(* Logix 5000 AddOnInstructionDefinition export PPD_IO_Link_Cyclic_Com_1_0_0; software revision 35.00 *)

ADD_ON_INSTRUCTION PPD_IO_Link_Cyclic_Com_1_0_0   (* revision 1.0 0, ExecutePrescan, ExecuteEnableInFalse *)
// FUNCTION_BLOCK PPD IO-Link Allen Breadley
VAR_INPUT
   in_b_RELEASE_FUNCTION_BLOCK : BOOL; {visible}
   in_b_00_FAST_STOP : BOOL; {visible}
   in_b_02_ACKNOLEDGE : BOOL; {visible}
   in_b_06_REPEAT_COMMAND_TOGGLE : BOOL; {visible}
   in_b_07_GRIP_DIRECTION : BOOL; {visible}
   in_b_08_JOG_MODE_NEGATIVE : BOOL; {visible}
   in_b_09_JOG_MODE_POSITIVE : BOOL; {visible}
   in_b_10_EXHAUST : BOOL; {visible}
   in_b_11_CALIBRATE : BOOL; {visible}
   in_b_16_MOVE_TO_ABSOLUTE_POSITION : BOOL; {visible}
   in_b_17_MOVE_TO_RELATIVE_POSITION : BOOL; {visible}
   in_b_18_FULLY_CLOSE : BOOL; {visible}
   in_b_19_FULLY_OPEN : BOOL; {visible}
   in_b_20_GRIP_WORKPIECE : BOOL; {visible}
   in_b_21_GRIP_WORKPIECE_AT_EXPECTED_POS : BOOL; {visible}
   in_b_22_CLOSE_ALL_VALVES : BOOL; {visible}
   in_usi_GAIN : USINT; {visible}
   in_usi_SPEED : USINT; {visible}
   in_ui_TARGET_POSITION_PRECICION : UINT; {visible}
   in_di_TARGET_POSITION : DINT; {visible}
   in_ui_TARGET_PRESSURE : UINT; {visible}
END_VAR
VAR_OUTPUT
   out_b_00_READY_FOR_OPERATION : BOOL; {access Read Only, visible}
   out_b_01_CONTOL_AUTHORITY_FIELDBUS : BOOL; {access Read Only, visible}
   out_b_03_NOT_FEASIBLE : BOOL; {access Read Only, visible}
   out_b_04_SENSOR_CALIBRATED : BOOL; {access Read Only, visible}
   out_b_05_COMMAND_RECEIVED_TOGGLE : BOOL; {access Read Only, visible}
   out_b_06_WARNING : BOOL; {access Read Only, visible}
   out_b_07_ERROR : BOOL; {access Read Only, visible}
   out_b_08_ALL_VALVES_CLOSED : BOOL; {access Read Only, visible}
   out_b_09_EXHAUSTED : BOOL; {access Read Only, visible}
   out_b_16_POSITION_REACHED : BOOL; {access Read Only, visible}
   out_b_17_NO_WORKPIECE_DETECTED : BOOL; {access Read Only, visible}
   out_b_18_WORKPIECE_GRIPPED : BOOL; {access Read Only, visible}
   out_b_19_WRONG_WORKPIECE_GRIPPED : BOOL; {access Read Only, visible}
   out_b_20_WORKPIECE_LOST : BOOL; {access Read Only, visible}
   out_usi_WARNING_CODE : USINT; {access Read Only, visible}
   out_usi_ERROR_CODE : USINT; {access Read Only, visible}
   out_di_ACTUAL_POSITION : DINT; {access Read Only, visible}
   out_i_ACTUAL_PRESSURE : INT; {access Read Only, visible}
END_VAR
VAR_IN_OUT
   in_PPD_PROZESS_DATA_IN : AB:PPD_XX_A4AF20E5:I:0; {required}
   out_PPD_PROZESS_DATA_OUT : AB:PPD_XX_88C23E22:O:0; {required}
END_VAR

ROUTINE EnableInFalse   (* structured text *)
   //////////////////////////////////////////////////////////////
   //   Copyright (c)  <Company Information>
   //--------------------------------------------------------------
   //   Routine: <Routine Name>
   //       Author: <Developer Name>
   //   Created: <Date>
   //--------------------------------------------------------------
   //   Description:
   //
   //   History:
   //
   /////////////////////////////////////////////////////////////
END_ROUTINE

ROUTINE Logic   (* structured text *)
   
   (*
   FUNCTION_BLOCK FB_SFP_EGU/EGK Allen Breadley
   TITLE = 'PPD_Cyclic_Communication'
   VERSION : '1.0.0'
   AUTHOR  : 'SCHUNK'
   NAME    : 'PPD_Cyclic_Communication'
   FAMILY  : 'SCHUNK'
   Used Products : PPD
   Projekt Nr.:
   =============================================================================
    Schunk GmbH&Co.KG
    (c)Copyright (2022) All Rights Reserved
   -----------------------------------------------------------------------------
    Library:       Schunk
    Tested with:   V35.00.00
                   Schunk FW release 5.x
    Engineering:   Studio 5000 V35.00.00
    Restrictions:  XXX(OB types, etc.)
    Requirements:  (hardware, technological package, memory needed, etc.)
    Functionality: The Funktion Block communicates Cyclic with the Gripper to read and wright Data
   
   *************************************************************************
   Historie
   
   ####################
   1.0.0
   Release Funktion Block
   TagType="Base" DataType="BOOL" Usage="Input" Radix="Binary" Required="false" Visible="true" ExternalAccess="Read Only"
   
   *************************************************************************)
   	(*English
   
       Statement section REGION
   
       *************************************************************************
       The function block is TO read AND transfer cyclic parameters that are changed FOR specific functions in the device
       can be used TO make The application process safer OR faster.
   
       Input parameters:
       ------------------
       b_RELEASE_FUNCTION_BLOCK            : Release FOR processing the block
   
       b_00_FAST_STOP                      : immediate shutdown of The process currently running in the gripper and shutdown of the motor phases
       b_02_ACKNOLEDGE                     : As long as the PPD is in error state and if an acknowledge was triggered, the PPD shall check if there are still any error causes.
                                             If there are no error causes any more, the state shall change to operational.
                                             Operational readiness is not established (again).
                                             If there are still any error causes, the status shall remain in error state and transmit the latest error code.
       b_06_REPEAT_COMMAND_TOGGLE          : The command that is still pending can, if it is a repeatable command, be repeated without loss OF Time for each positive and negative change of this bit
       b_07_GRIP_DIRECTION                 : determines The gripping direction. FALSE = external gripping (the workpiece is gripped from the outside) / True = internal gripping (the workpiece is gripped from the inside).
   
       b_08_JOG_MODE_NEGATIVE              : The gripper shall execute a movement with a fix velocity in the control bit corresponding direction.
                                             The value of the used fix velocity shall be 1 mm/s.
                                             Negative means a movement in the direction of decreasing position values. Function is also possible without "Calibration".
       b_09_JOG_MODE_POSITIVE              : The gripper shall execute a movement with a fix velocity in the control bit corresponding direction.
                                             The value of the used fix velocity shall be 1 mm/s.
                                             Positive means a movement in the direction of increasing position values. Function is also possible without "Calibration".
       b_10_EXHAUST                        : As soon as this function has been triggered the PPD shall open all valves to exhaust the air of both chambers.
                                             To trigger this function the PPD shall be in operation or error status.
       b_11_CALIBRATE                      : The calibrate function creates a routine in the PPD that determines the minimum and maximum position of the connected pneumatic product,
                                             provided a measuring system is available. The routine runs automatically.
   
       b_16_MOVE_TO_ABSOLUTE_POSITION      : When executing the command, the PPD tries to move to the specified position "Tag Position".
                                             In order to be able to execute this function, further parameters must be transferred: target accuracy, speed, gain.
       b_17_MOVE_TO_RELATIVE_POSITION      : When the command is executed, the PPD attempts to move to the specified, calculated position.
                                             In order to be able to execute this function, further parameters must be transferred: target position, target accuracy, speed, gain.
       b_18_FULLY_CLOSE                    : With this function, the PPD executes a movement to the minimum possible position.
       b_18_FULLY_OPEN                     : With this function, the PPD executes a movement to the maximum possible position.
       b_20_GRIP_WORKPIECE                 : The gripper shall grip workpieces at a nonspecific position.
                                             To execute this function the following parameter values shall be transmitted.
                                                   - target pressure difference
                                                   - speed
                                                   - grip direction (control bit)
       b_21_GRIP_WORKPIECE_AT_EXPECTED_POSITION : The gripper should grip workpieces at a specific position.
                                                  To execute this function, the following parameter values must be transferred.
                                                        - target position
                                                        - target pressure difference
                                                        - speed
       b_22_CLOSE_ALL_VALVES               : As soon as this function has been triggered the PPD shall close all valves.
   
       usi_GAIN                            : If a function needs a gain value to execute, the IO-Link master must transfer this value in the cyclic gain parameter.
                                             The gain value ranges from 1 to 10
       usi_SPEED                           : If a function needs a speed value to execute, the IO-Link-Master shall transmit this value in the cyclic parameter speed.
                                             Valid values shall be 1 to 10.
       i_TARGET_POSITION_PRECICION         : The parameter must represent a value in micrometers [µm].
                                             Valid values are between 500 µm and 15,000 µm.
       di_TARGET_POSITION                  : Valid values shall be -5.000.000 µm to 5.000.000 µm.
       ui_TARGET_PRESSURE			        : The target pressure difference shall represent the mathematical absolute value of the pressure difference between the two compression chambers.
                                             Valid values shall be 2000 mbar to 8.000 mbar.
   
       #################
   
   
   
       Output parameters:
       ------------------
   
       b_00_READY_FOR_OPERATION            : indicates that the gripper is ready FOR operation
       b_01_CONTOL_AUTHORITY_FIELDBUS      : indicates whether the fieldbus has control authority over the gripper
       b_03_NOT_FEASIBLE                   : Indicates that the last issued command cannot be executed.
                                               Possible causes are:
                                               - a new command was sent although the command that is still active has NOT yet been processed.
                                               - 2 OR more control commands simultaneously active in the control word
                                               - Parameter data FOR position, speed OR force are outside the permissible limits.
   
       b_04_SENSOR_CALIBRATED              : indicates that the "Calibrate" command was executed correctly and the sensor is calibrated
       b_05_COMMAND_RECEIVED_TOGGLE        : indicates that a command was sent to The gripper via the bus. the command does not have TO be processed or started at the time it is displayed.
       b_06_WARNING                        : signals a warning in the gripper, e.g. temperature warning
       b_07_ERROR                          : signals a fault in the gripper, e.g. rapid stop
       b_08_ALL_VALVES_CLOSED              : indicates that all Valves are closed
       b_09_EXHAUSTED                      : indicates that the EXHAUST funktion is completed successfully
   
       b_16_POSITION_REACHED               : signals that the relative or absolute position has been approached
       b_17_NO_WORKPIECE_DETECTED          : indicates that no workpiece was detected
       b_18_WORKPIECE_GRIPPED              : signals that a workpiece has been gripped
       b_19_WRONG_WORKPIECE_DETECTED       : signals that a wrong workpiece was detected
       b_20_WORKPIECE_LOST                 : signals that the gripped workpiece was lost
   
       usi_WARNING_CODE                     : Output of the gripper's warning code
       usi_ERROR_CODE                       : Output of the error code of the gripper
   
       di_ACTUAL_POSITION                  : the current position OF The gripper is returned here
       i_ACTUAL_PRESSURE_DIFFERENCE        : As long as a workpiece is being gripped, the IO-Link master should be able to evaluate the actual signed pressure difference value by reading out the cyclic parameter actual pressure difference.
                                             The value is shown in millibar [mbar].
   
       *************************************************************************)
   
   
   (*************************************************************************
       Der Baustein soll Zyklische Parameter einlesen und übertragen, welche für bestimmte Funktionen im Gerät geändert
       werden können um den Applikationsprozess sicherer oder schneller zu machen.
   
       Eingangsparameter:
       ------------------
   
       b_RELEASE_FUNCTION_BLOCK            : Freigabe zur Bearbeitung des Bausteins (True = Freigabe zur Bearbeitung)
   
       b_00_FAST_STOP                      : Sobald diese Funktion ausgelöst wird, wird jede Bewegung abgebrochen und der PPD in den Fehlerzustand versetzt.
       b_02_ACKNOLEDGE                     : Solange sich das PPD im Fehlerzustand befindet und eine Bestätigung ausgelöst wurde, prüft das PPD, ob noch Fehlerursachen vorliegen.
                                             Liegen keine Fehlerursachen mehr vor, wechselt der Zustand in „Operational“.
                                             Die Betriebsbereitschaft ist nicht (wieder) hergestellt.
                                             Liegen weiterhin Fehlerursachen vor, bleibt der Status im Fehlerzustand und übermittelt den aktuellsten Fehlercode.
       b_06_REPEAT_COMMAND_TOGGLE          : Das Noch anstehende Kommando kann, sofern es ein wiederholbares Kommando ist, ohne Zeitverlust bei jedem positiven und negativen Wechsel dieses Bits wiederholt werden
       b_07_GRIP_DIRECTION                 : legt die Greifrichtung fest. FALSE = Ausengreifen (Das Werkstück wird von außen gegriffen) / True = Innengreifen (Das Werkstück wird von innen gegriffen).
   
       b_08_JOG_MODE_NEGATIVE              : Der Greifer soll eine Bewegung mit fester Geschwindigkeit in die dem Steuerbit entsprechende Richtung ausführen.
                                             Der Wert der verwendeten Fixgeschwindigkeit muss 1 mm/s betragen.
                                             Negativ bedeutet eine Bewegung in Richtung abnehmender Positionswerte. Funktion ist auch ohne „Kalibrierung“ möglich.
       b_09_JOG_MODE_POSITIVE              : Der Greifer soll eine Bewegung mit fester Geschwindigkeit in die dem Steuerbit entsprechende Richtung ausführen.
                                             Der Wert der verwendeten Fixgeschwindigkeit muss 1 mm/s betragen.
                                             Positiv bedeutet eine Bewegung in Richtung steigender Positionswerte. Funktion ist auch ohne „Kalibrierung“ möglich.
       b_10_EXHAUST                        : Sobald diese Funktion ausgelöst wurde, öffnet die PPD alle Ventile, um die Luft aus beiden Kammern abzulassen.
                                             Um diese Funktion auszulösen, muss sich die PPD im Betriebs- oder Fehlerstatus befinden.
       b_11_CALIBRATE                      : Die Funktion Kalibrieren stertet in der PPD eine Rutiene welche die minimale und maximale Position der angeschlossenen Pneumatischen produktes ermittelt,
                                             sofern ein Messsystem vorhanden ist. Die Routine läuft selbständig ab.
   
       b_16_MOVE_TO_ABSOLUTE_POSITION      : Beim ausführen des Befehls versucht die PPD aud die vorgegebene Position "Taget Position" zu fahren.
                                             Um diese Funktion ausführen zu können, müssen weitere Parameter übertragen werden: target accurancy, Speed, Gain
       b_17_MOVE_TO_RELATIVE_POSITION      : Beim ausführen des Befehls versucht die PPD auf die vorgegebene errechnete Position zu fahren.
                                             Um diese Funktion ausführen zu können, müssen weitere Parameter übertragen werden: target possition, target accurancy, Speed, Gain.
       b_18_FULLY_CLOSE                    : Bei dieser Funktion führt die PPD eine Bewegung auf die minimal mögliche Position aus.
       b_19_FULLY_OPEN                     : Bei dieser Funktion führt die PPD eine Bewegung auf die maximal mögliche Position aus.
       b_20_GRIP_WORKPIECE                 : Der Greifer soll Werkstücke an einer unbestimmten Position greifen.
                                             Zur Ausführung dieser Funktion müssen folgende Parameterwerte übertragen werden.
                                                   - target pressure difference
                                                   - speed
                                                   - grip direction (control bit)
   
       b_21_GRIP_WORKPIECE_AT_EXPECTED_POSITION    : Der Greifer soll Werkstücke an einer bestimmten Position greifen.
                                                     Zur Ausführung dieser Funktion müssen folgende Parameterwerte übertragen werden.
                                                           - target position
                                                           - target pressure difference
                                                           - speed
       b_22_CLOSE_ALL_VALVES               : Sobald diese Funktion ausgelöst wurde, soll das PPD alle Ventile schließen.
   
   
       usi_GAIN                            : Wenn eine Funktion zur Ausführung einen Verstärkungswert benötigt, muss der IO-Link-Master diesen Wert im zyklischen Parameter Verstärkung übertragen.
                                             Der Wert der Verstärkung bewegt sich zwischen 1 und 10
       usi_SPEED                           : Benötigt eine Funktion zur Ausführung einen Geschwindigkeitswert, muss der IO-Link-Master diesen Wert im zyklischen Parameter Geschwindigkeit übertragen.
                                             Gültige Werte liegen zwischen 1 und 10.
       i_TARGET_POSITION_PRECICION         : Der Parameter muss einen Wert in Mikrometern [µm] darstellen.
                                             Gültige Werte liegen zwischen 500 µm und 15.000 µm.
       di_TARGET_POSITION                  : Gültige Werte liegen zwischen -5.000.000 µm und 5.000.000 µm.
       ui_TARGET_PRESSURE			        : Die Zieldruckdifferenz soll den mathematischen Absolutwert der Druckdifferenz zwischen den beiden Kompressionskammern darstellen.
                                             Gültige Werte liegen zwischen 2000 mbar und 8.000 mbar.
   
       ##################
   
   
       Ausgangsparameter:
       ------------------
   
       b_00_READY_FOR_OPPERATION           : zeigt die Betriebsbereitschaft des Greifers an
       b_01_CONTOL_AUTHORITY_FIELDBUS      : zeigt an, ob der Feldbus die Steuerhoheit über den Greifer hat
       b_03_NOT_FEASIBLE                   : Zeigt an, das der zuletzt abgesetzte Befehl nicht ausgeführt werden kann.
                                               Mögliche Ursachen sind:
                                               - ein neuer Befehl wurde abgesetzt, obwohl der noch aktive Befehl noch nicht abgearbeitet wurde.
                                               - 2 oder mehr Steuerbefehle gleichzeitig aktiv im Steuerwort
                                               - Parameterdaten von Position, Geschwindigkeit oder Kraft liegen auserhalb der Zulässigen grenzen.
   
       b_04_SENSOR_CALIBRATED              : Zeigt an das der Befehl "Calibrate" korrekt ausgeführt wurde und der Sensor Kalibriert ist
       b_05_COMMAND_RECEIVED_TOGGLE        : Zeigt an das ein Befehl über den Bus an den Greufer gesendet wurde. Zum Zeitpunkt der Anzeige muß der Befehl noch nicht abgearbeitet oder gestartet sein.
       b_06_WARNING                        : signalisiert eine Warnung im Greifer, z.B. Temperaturwarnung
       b_07_ERROR                          : signalisiert eine Störung im Greifer, z.B. Schnellstop
       b_08_ALL_VALVES_CLOSED              : zeigt an, dass alle Ventile geschlossen sind
       b_09_EXHAUSTED                      : zeigt an, dass die EXHAUST-Funktion erfolgreich abgeschlossen wurde
   
       b_16_POSITION_REACHED               : signalisiert, dass die relative oder absolute Position angefahren wurde
       b_17_NO_WORKPIECE_DETECTED          : signalisiert, dass kein Werkstück erkannt wurde
       b_18_WORKPIECE_GRIPPED              : signalisiert, dass ein Werkstück gegriffen wurde
       b_19_WRONG_WORKPIECE_DETECTED       : signalisiert, das ein falsches Werkstück erkannt wurde
       b_20_WORKPIECE_LOST                 : signalisiert, dass das gegriffene Werkstück verloren ging
   
       usi_WARNING_CODE                    : Ausgabe des Warnungscodes des Greifers
       usi_ERROR_CODE                      : Ausgabe des Störungscodes des Greifers
       di_ACTUAL_POSITION                  : hier wird die aktuelle Possition des Greifers zurückgegeben
       i_ACTUAL_PRESSURE_DIFFERENCE        : Solange ein Werkstück gegriffen wird, soll der IO-Link-Master in der Lage sein, den tatsächlichen vorzeichenbehafteten Druckdifferenzwert durch Auslesen des zyklischen Parameters Ist-Druckdifferenz auszuwerten.
                                             Der Wert wird in millibar [mbar] dargestellt.
   
   *************************************************************************)
   
       IF NOT in_b_RELEASE_FUNCTION_BLOCK
   
       THEN
   
   	out_PPD_PROZESS_DATA_OUT.fast_stop 									:= 0;
   	out_PPD_PROZESS_DATA_OUT.acknowledge 								:= 0;
   	//in_OUTPUT_DATA.repeat_command_toggle						:= 0;
   	//in_OUTPUT_DATA.grip_direction								:= 0;
   	out_PPD_PROZESS_DATA_OUT.jog_mode_negative							:= 0;
   	out_PPD_PROZESS_DATA_OUT.jog_mode_positive							:= 0;
   	out_PPD_PROZESS_DATA_OUT.exhaust										:= 0;
   	out_PPD_PROZESS_DATA_OUT.calibrate									:= 0;
   	out_PPD_PROZESS_DATA_OUT.move_to_absolute_position					:= 0;
   	out_PPD_PROZESS_DATA_OUT.move_to_relative_position					:= 0;
   	out_PPD_PROZESS_DATA_OUT.fully_closed								:= 0;
   	out_PPD_PROZESS_DATA_OUT.fully_open									:= 0;
   	out_PPD_PROZESS_DATA_OUT.grip_workpiece								:= 0;
   	out_PPD_PROZESS_DATA_OUT.grip_workpiece_at_expected_position			:= 0;
   	out_PPD_PROZESS_DATA_OUT.close_all_valves							:= 0;
   
   	out_PPD_PROZESS_DATA_OUT.gain										:= 0;
   	out_PPD_PROZESS_DATA_OUT.speed										:= 0;
   	out_PPD_PROZESS_DATA_OUT.target_accuracy								:= 0;
   	out_PPD_PROZESS_DATA_OUT.target_position								:= 0;
   	out_PPD_PROZESS_DATA_OUT.target_pressure_difference					:= 0;
   
   	TND( ); // Temp End
   
       END_IF;
   
   	// Read the Cyclic Date
   	// Einlesen der Zyklischen Daten
   
       // Enter the input data in the instance DB and assign them to the status displays
       // Eingangsdaten in den Instanz DB eintragen und den Statusanzeigen zuweisen
   
   	out_b_00_READY_FOR_OPERATION 				:= in_PPD_PROZESS_DATA_IN.ready_for_operation;
   	out_b_01_CONTOL_AUTHORITY_FIELDBUS 			:= in_PPD_PROZESS_DATA_IN.control_authority_fieldbus;
   
   	out_b_03_NOT_FEASIBLE 						:= in_PPD_PROZESS_DATA_IN.not_feasible;
   	out_b_04_SENSOR_CALIBRATED					:= in_PPD_PROZESS_DATA_IN.sensor_calibrated;
   	out_b_05_COMMAND_RECEIVED_TOGGLE 			:= in_PPD_PROZESS_DATA_IN.command_received_toggle;
   	out_b_06_WARNING 							:= in_PPD_PROZESS_DATA_IN.warning;
   	out_b_07_ERROR 								:= in_PPD_PROZESS_DATA_IN.error;
   	out_b_08_ALL_VALVES_CLOSED			 		:= in_PPD_PROZESS_DATA_IN.all_valves_closed;
   	out_b_09_EXHAUSTED 							:= in_PPD_PROZESS_DATA_IN.actuator_exhausted;
   
   	out_b_16_POSITION_REACHED 					:= in_PPD_PROZESS_DATA_IN.position_reached;
   	out_b_17_NO_WORKPIECE_DETECTED 				:= in_PPD_PROZESS_DATA_IN.no_workpiece_detected;
   	out_b_18_WORKPIECE_GRIPPED					:= in_PPD_PROZESS_DATA_IN.workpiece_lost;
   	out_b_19_WRONG_WORKPIECE_GRIPPED			:= in_PPD_PROZESS_DATA_IN.wrong_workpiece_gripped;
   	out_b_20_WORKPIECE_LOST						:= in_PPD_PROZESS_DATA_IN.workpiece_lost;
   
   	out_usi_WARNING_CODE						:= in_PPD_PROZESS_DATA_IN.warning_code;
   	out_usi_ERROR_CODE							:= in_PPD_PROZESS_DATA_IN.error_code;
   	out_di_ACTUAL_POSITION						:= in_PPD_PROZESS_DATA_IN.actual_position;
   	out_i_ACTUAL_PRESSURE						:= in_PPD_PROZESS_DATA_IN.actual_pressure_difference;
   
       // Allocation of output data for the periphery
       // Zuweisung der Ausgangsdaten für die Peripher
   
   
   	out_PPD_PROZESS_DATA_OUT.fast_stop								:= in_b_00_FAST_STOP;
   	out_PPD_PROZESS_DATA_OUT.acknowledge							:= in_b_02_ACKNOLEDGE;
   	out_PPD_PROZESS_DATA_OUT.repeat_toggle_command					:= in_b_06_REPEAT_COMMAND_TOGGLE;
   	out_PPD_PROZESS_DATA_OUT.grip_direction							:= in_b_07_GRIP_DIRECTION;
   	out_PPD_PROZESS_DATA_OUT.jog_mode_negative						:= in_b_08_JOG_MODE_NEGATIVE;
   	out_PPD_PROZESS_DATA_OUT.jog_mode_positive						:= in_b_09_JOG_MODE_POSITIVE;
   	out_PPD_PROZESS_DATA_OUT.exhaust								:= in_b_10_EXHAUST;
   	out_PPD_PROZESS_DATA_OUT.calibrate								:= in_b_11_CALIBRATE;
   
   	out_PPD_PROZESS_DATA_OUT.move_to_absolute_position				:= in_b_16_MOVE_TO_ABSOLUTE_POSITION;
   	out_PPD_PROZESS_DATA_OUT.move_to_relative_position				:= in_b_17_MOVE_TO_RELATIVE_POSITION;
   	out_PPD_PROZESS_DATA_OUT.fully_closed							:= in_b_18_FULLY_CLOSE;
   	out_PPD_PROZESS_DATA_OUT.fully_open								:= in_b_19_FULLY_OPEN;
   	out_PPD_PROZESS_DATA_OUT.grip_workpiece							:= in_b_20_GRIP_WORKPIECE;
   	out_PPD_PROZESS_DATA_OUT.grip_workpiece_at_expected_position	:= in_b_21_GRIP_WORKPIECE_AT_EXPECTED_POS;
   	out_PPD_PROZESS_DATA_OUT.close_all_valves						:= in_b_22_CLOSE_ALL_VALVES;
   
   	out_PPD_PROZESS_DATA_OUT.gain									:= in_usi_GAIN;
   	out_PPD_PROZESS_DATA_OUT.speed									:= in_usi_SPEED;
   	out_PPD_PROZESS_DATA_OUT.target_accuracy						:= in_ui_TARGET_POSITION_PRECICION;
   	out_PPD_PROZESS_DATA_OUT.target_position						:= in_di_TARGET_POSITION;
   	out_PPD_PROZESS_DATA_OUT.target_pressure_difference				:= in_ui_TARGET_PRESSURE;
   
END_ROUTINE

ROUTINE Postscan   (* structured text *)
   //////////////////////////////////////////////////////////////
   //   Copyright (c)  <Company Information>
   //--------------------------------------------------------------
   //   Routine: <Routine Name>
   //       Author: <Developer Name>
   //   Created: <Date>
   //--------------------------------------------------------------
   //   Description:
   //
   //   History:
   //
   /////////////////////////////////////////////////////////////
END_ROUTINE

ROUTINE Prescan   (* structured text *)
   //////////////////////////////////////////////////////////////
   //   Copyright (c)  <Company Information>
   //--------------------------------------------------------------
   //   Routine: <Routine Name>
   //       Author: <Developer Name>
   //   Created: <Date>
   //--------------------------------------------------------------
   //   Description:
   //
   //   History:
   //
   /////////////////////////////////////////////////////////////
END_ROUTINE
END_ADD_ON_INSTRUCTION
